TYPE ST_SentRawNibbleData :
STRUCT
	nStatusTicks		: USINT;
	nNibbleTicks		: ARRAY[1..6] OF USINT;
	nCrcTicks			: USINT;
	
	nStatusValue		: USINT;
	nNibbleValue		: ARRAY[1..6] OF USINT;
	nCrcValue			: USINT; 
END_STRUCT
END_TYPE
